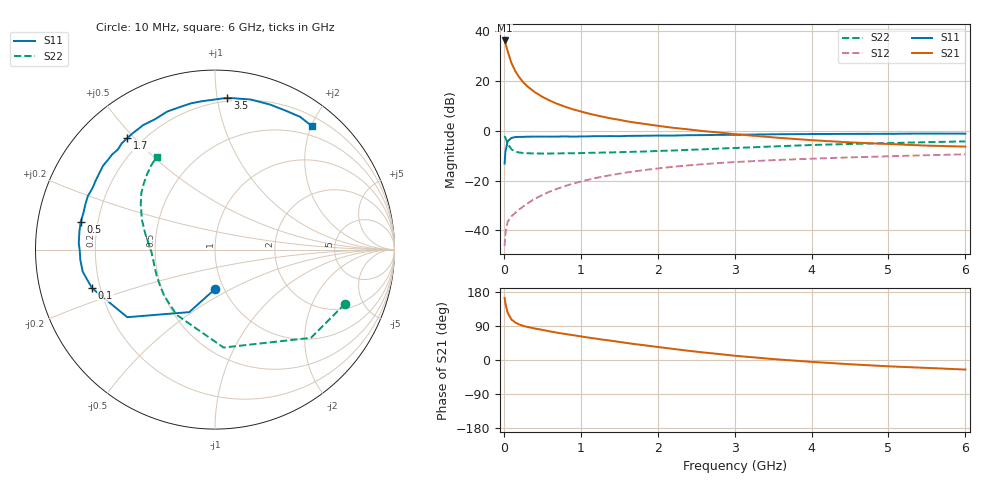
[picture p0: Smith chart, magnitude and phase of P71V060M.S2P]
! SIEMENS Small Signal Semiconductors
! BFP196
! Si NPN RF Bipolar Junction Transistor in SOT143
! VCE = 1 V  IC = 60 mA
! Common Emitter S-Parameters:  May  1996
# GHz  S  MA  R  50
!  f  S11  S21  S12  S22
! GHz  MAG  ANG  MAG  ANG  MAG  ANG  MAG  ANG
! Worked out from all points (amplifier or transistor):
!   36 points, 10 MHz to 6 GHz, reference 50 ohm
!   highest |S21| = 36.3 dB at 10 MHz (marker M1)
!   |S21| within 3 dB of that: start of sweep to 37.91 MHz
!   unconditionally stable (mu >= 1): 331.5 MHz to end of sweep
!   at 250 MHz: K = 0.94, MSG = 25.0 dB, |S12| = -30.5 dB
!   at 1.4 GHz: K = 1.11, MAG = 9.3 dB, |S12| = -17.8 dB
!   at 6 GHz: K = 1.03, MAG = 0.6 dB, |S12| = -9.5 dB
!   S11 on the Smith chart (normalised r, x): 10 MHz: 0.91, -0.42; 100 MHz: 0.17, -0.15; 500 MHz: 0.14, +0.10; 1.7 GHz: 0.14, +0.48; 3.5 GHz: 0.18, +1.07; 6 GHz: 0.34, +2.01
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0.01  0.2184 -89.6  65.19 164.2  0.0048 72.9  0.7849 -22.6
0.02  0.3768 -112.4  58.62 149.8  0.0086 64.2  0.7262 -42.6
0.05  0.6172 -142.4  39.27 124.3  0.0149 47.9  0.5477 -85.0
0.1  0.718 -162.6  22.72 106.7  0.0191 46.4  0.4217 -120.5
0.15  0.7472 -170.5  15.64 98.8  0.0226 49.4  0.3824 -137.8
0.2  0.7526 -175.7  11.89 93.8  0.0264 52.7  0.3649 -147.6
0.25  0.7535 -179.6  9.486 90.3  0.0299 55.7  0.3575 -154.4
0.3  0.7597 177.3  7.941 87.6  0.0342 58.3  0.3535 -158.6
0.4  0.7624 172.2  6.006 83.2  0.0427 61.3  0.3499 -164.7
0.5  0.7638 168.3  4.811 79.5  0.0511 62.9  0.3488 -168.7
0.6  0.761 164.3  4.011 75.5  0.0602 63.7  0.3489 -171.5
0.7  0.7654 160.4  3.448 71.7  0.069 63.4  0.3508 -173.8
0.9  0.7637 153.5  2.693 65.5  0.087 61.9  0.3531 -177.4
1.1  0.7721 146.9  2.223 59.2  0.104 59.8  0.3595 179.9
1.3  0.7783 139.9  1.893 53.3  0.1214 57.0  0.3644 177.3
1.7  0.7902 128.1  1.462 42.0  0.1527 51.2  0.378 172.4
2.2  0.7998 114.6  1.146 29.3  0.1888 43.4  0.4012 166.4
3  0.8298 95.1  0.856 11.3  0.235 30.9  0.4501 155.3
3.5  0.8487 85.3  0.736 2.5  0.2567 23.8  0.484 148.7
4.5  0.8643 69.3  0.584 -11.2  0.2919 11.6  0.5425 136.9
5.5  0.8788 57.3  0.503 -20.9  0.3225 0.8  0.5894 127.0
6  0.8745 51.8  0.48 -25.2  0.3362 -5.0  0.6112 122.0
